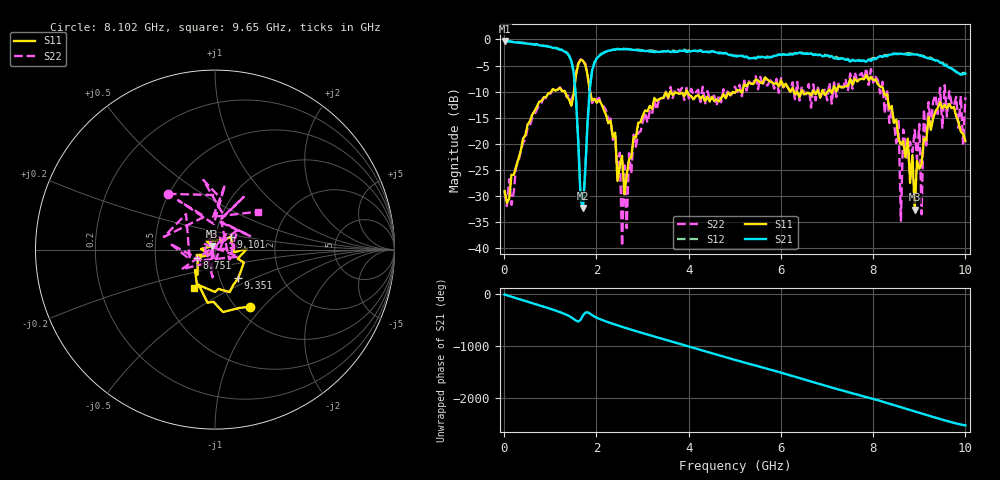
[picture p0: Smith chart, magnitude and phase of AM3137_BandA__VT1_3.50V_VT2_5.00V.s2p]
! Date/Time: Tue, Nov 13, 2018 4:48 PM
! Network Analyzer: Agilent Technologies E8364B Rev: A.07.50.67
! Sweep from 0.010 to 10.000 GHz, 201 Points, Sweep Type: LIN
! Power Supply: 3.501 V, -0.003 A
# Hz S DB R 50
!freq MagS11 AngS11 MagS21 AngS21 MagS12 AngS12 MagS22 AngS22
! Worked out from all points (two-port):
!   201 points, 10 MHz to 10 GHz, reference 50 ohm
!   highest |S21| = -0.29 dB at 10 MHz (marker M1); lowest = -32.3 dB at 1.708 GHz (marker M2)
!   |S21| within 3 dB of the highest: start of sweep to 1.416 GHz; 2.047 GHz to 5.184 GHz (3.137 GHz wide, 86.8 % of centre)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
!   lowest |S11| = -32.6 dB at 8.901 GHz (marker M3), VSWR 1.05, Z = 48.5 + j1.74 ohm
!   |S11| at or under -10 dB: 1.858 GHz to 3.601 GHz (1.743 GHz wide, 63.8 % of centre); 3.971 GHz to 5.025 GHz (1.054 GHz wide, 23.4 % of centre); 8.23 GHz to end of sweep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
!   |S22| runs from -39.6 to -3.8 dB; largest |S21 - S12| = 0.038
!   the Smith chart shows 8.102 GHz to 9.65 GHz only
!   S11 on the Smith chart (normalised r, x): 8.102 GHz: 1.15, -0.85; 8.751 GHz: 0.81, -0.07; 9.101 GHz: 1.18, +0.17; 9.351 GHz: 1.22, -0.41; 9.65 GHz: 0.73, -0.33
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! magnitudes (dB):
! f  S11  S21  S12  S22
! 10 MHz  -29.0  -0.3  -0.2  -29.3
! 1.409 GHz  -11.6  -3.1  -3.1  -10.6
! 1.708 GHz  -4.1  -32.3  -32.2  -4.2
! 1.908 GHz  -11.7  -5.9  -5.8  -12.2
! 2.508 GHz  -24.1  -1.9  -1.8  -21.7
! 2.557 GHz  -22.3  -1.9  -1.8  -39.6
! 2.607 GHz  -29.7  -1.9  -1.8  -24.1
! 3.357 GHz  -11.4  -2.4  -2.4  -11.5
! 5.005 GHz  -10.2  -3.2  -3.1  -9.0
! 6.703 GHz  -9.8  -3.0  -2.9  -8.6
! 8.102 GHz  -8.6  -3.4  -3.5  -7.8
! 8.352 GHz  -13.3  -2.9  -2.7  -16.0
! 8.551 GHz  -19.1  -2.8  -2.8  -15.6
! 8.601 GHz  -20.1  -2.7  -2.8  -34.7
! 8.651 GHz  -19.5  -2.8  -2.8  -17.2
! 8.751 GHz  -19.0  -2.9  -2.6  -23.2
! 8.901 GHz  -32.6  -2.9  -2.9  -17.3
! 9.051 GHz  -23.8  -3.1  -3.0  -33.5
! 9.101 GHz  -19.0  -3.4  -3.2  -13.3
! 9.351 GHz  -13.7  -4.0  -4.1  -10.6
! 9.65 GHz  -12.3  -5.4  -5.3  -9.9
! 10 GHz  -19.4  -6.5  -6.4  -11.1
